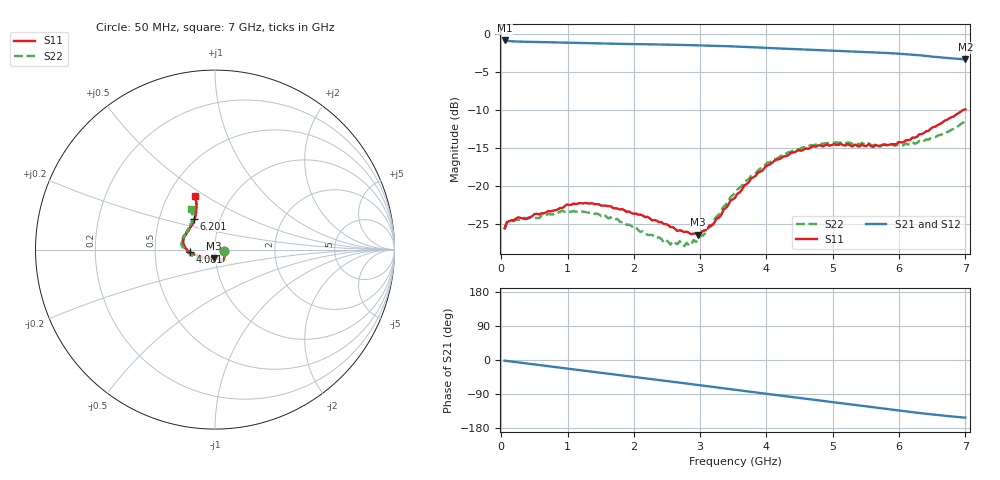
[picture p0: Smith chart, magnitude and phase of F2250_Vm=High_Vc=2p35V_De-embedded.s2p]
! Integrated Device Technology
! Corporate Headquarters
! 6024 Silver Creek Valley Road
! San Jose, CA 95138  USA
! Phone:  1-408-284-8200
! Toll Free:  1-800-223-1366
! Webpage:  http://www.idt.com/
! Timing and RF Division
! 515 Groton Road, Suite 102
! Westford, MA 01886-6024
! Device:  F2250
! Description: Voltage Variable RF Attenuator
! Frequency:  50.0 -  6000.00 MHz
! Package:  3x3 mm Thin QFN Plastic Package: 16 pin
! Ports:  2 RF, 3 DC
!  Pin  1  = GND
!  Pin  2  = NC
!  Pin  3  = RF1  = Port 1
!  Pin  4  = NC
!  Pin  5  = GND
!  Pin  6  = GND
!  Pin  7  = GND
!  Pin  8  = GND
!  Pin  9  = NC
!  Pin 10  = RF2  = Port 2
!  Pin 11  = NC
!  Pin 12  = GND
!  Pin 13  = GND
!  Pin 14  = VCNTRL
!  Pin 15  = VDD
!  Pin 16  = VMODE
! Vcntrl:  2.350 Volts
! Vmode:  +3.300 Volts
! Vdd:  +3.30  Volts
! Current:  1.316 mA
! Data:  The device was measured on a the F2250 evaluation board which has
!  individual transmission lines to the RF pins.  Data was collected
!  using a calibrated network analyzer.  The evaluation board was
!  de-embedded using a TRL calibration technique.
!  The reference plane is the edge of the package pin.
! Misc:  SN 10
!  Action Tracker AT0258
! Date Measured:  2014-11-26
! Date:  2015-10-15  MJV
! Note:
!  Integrated Device Technology supplies this data as a sample of measured
!  data at the package pin for this product.  Your particular data for this
!  product may vary.
!  Data was taken at 25 degrees C.
!  Integrated Device Technology reserves the right to change this data at anytime.
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# GHz S dB R 50
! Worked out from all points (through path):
!   201 points, 50 MHz to 7 GHz, reference 50 ohm
!   highest |S21| = -0.90 dB at 50 MHz (marker M1); lowest = -3.4 dB at 7 GHz (marker M2)
!   group delay of S21, straight-line fit = 61.2 ps
!   lowest |S11| = -26.4 dB at 2.969 GHz (marker M3), VSWR 1.10, Z = 49.2 - j4.68 ohm
!   |S11| at or under -10 dB: start of sweep to 6.974 GHz
!   |S22| runs from -27.9 to -11.5 dB; largest |S21 - S12| = 0.0019
!   S11 on the Smith chart (normalised r, x): 50 MHz: 1.11, -0.02; 4.081 GHz: 0.75, -0.02; 6.201 GHz: 0.75, +0.27; 7 GHz: 0.68, +0.45
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0.05  -25.53 -10.5  -0.90 -1.8  -0.90 -1.8  -25.69 -10.8
0.1195  -24.63 -10.1  -0.99 -3.2  -0.99 -3.2  -24.57 -8.8
0.57125  -23.73 -31.1  -1.11 -13.3  -1.11 -13.3  -24.22 -31.2
0.91875  -22.91 -49.7  -1.18 -21.0  -1.18 -21.1  -23.26 -50.8
1.2315  -22.28 -57.5  -1.25 -27.9  -1.25 -27.9  -23.37 -61.3
1.75275  -22.95 -64.4  -1.34 -39.1  -1.34 -39.1  -24.31 -67.7
2.37825  -24.75 -64.2  -1.43 -52.8  -1.43 -52.8  -26.73 -67.0
2.552  -25.39 -69.1  -1.45 -56.7  -1.45 -56.7  -27.70 -73.4
2.691  -25.81 -77.0  -1.48 -59.8  -1.48 -59.8  -27.23 -81.1
2.7605  -26.05 -79.2  -1.49 -61.3  -1.49 -61.3  -27.90 -85.6
2.969  -26.40 -97.1  -1.53 -66.0  -1.53 -66.0  -27.14 -104.9
3.1775  -25.17 -120.1  -1.58 -70.7  -1.58 -70.7  -25.14 -126.6
3.525  -21.55 -152.2  -1.69 -78.5  -1.69 -78.6  -20.92 -148.6
3.76825  -18.99 -164.4  -1.78 -84.0  -1.78 -84.1  -18.66 -159.6
4.081  -16.97 -175.4  -1.91 -91.0  -1.91 -91.0  -16.69 -171.4
4.4285  -15.55 176.2  -2.04 -98.6  -2.04 -98.7  -15.18 178.7
4.7065  -14.78 169.3  -2.14 -104.8  -2.14 -104.8  -14.67 173.0
5.054  -14.62 161.1  -2.27 -112.5  -2.26 -112.5  -14.27 166.0
5.85325  -14.59 135.2  -2.57 -130.0  -2.57 -130.1  -14.68 147.2
6.20075  -13.64 123.7  -2.77 -137.7  -2.78 -137.8  -14.25 138.2
6.54825  -12.21 115.7  -3.05 -144.7  -3.05 -144.9  -13.59 126.9
7  -9.93 110.9  -3.37 -152.1  -3.38 -152.2  -11.55 120.7
